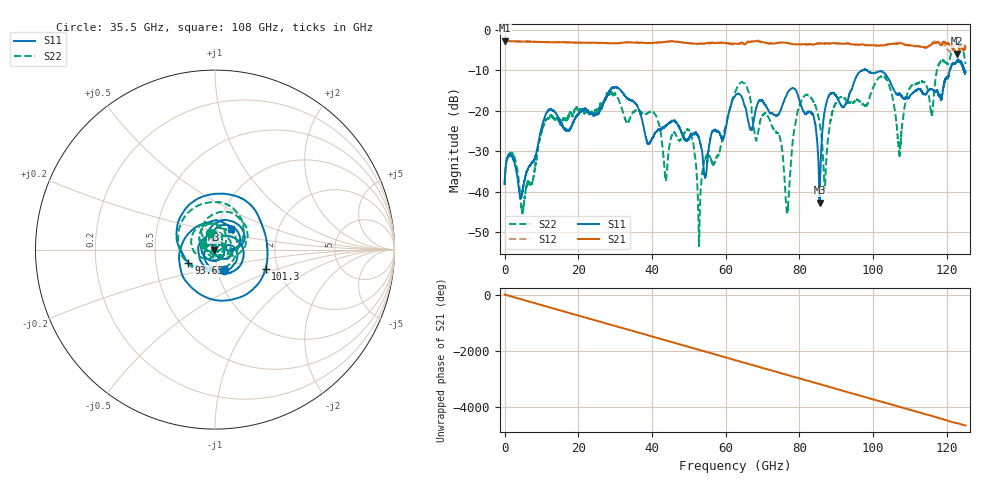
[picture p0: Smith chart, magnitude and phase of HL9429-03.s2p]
! 1/9/2024 4:34:33 PM
! H:\PROTOTYPE_DATA\110GHZ-ATTN\3DB\3089.S2P
! CHANNEL.1
! TR.MEASUREMENT
! CORRECTED.DATA
# GHZ S RI R 50.0
! FREQ.GHZ  S11RE  S11IM  S21RE  S21IM  S12RE  S12IM  S22RE  S22IM
!; PortSelection: Port_12
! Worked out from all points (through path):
!   5000 points, 25 MHz to 125 GHz, reference 50 ohm
!   highest |S21| = -2.70 dB at 25 MHz (marker M1); lowest = -5.9 dB at 122.8 GHz (marker M2)
!   group delay of S21, straight-line fit = 104 ps
!   lowest |S11| = -42.7 dB at 85.45 GHz (marker M3), VSWR 1.01, Z = 49.3 - j0.0201 ohm
!   |S11| at or under -10 dB: start of sweep to 97.18 GHz; 98.2 GHz to 120.8 GHz (22.57 GHz wide, 20.6 % of centre); 124.5879 GHz to end of sweep
!   |S22| runs from -53.5 to -2.9 dB; largest |S21 - S12| = 0.23
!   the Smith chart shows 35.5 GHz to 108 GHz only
!   S11 on the Smith chart (normalised r, x): 35.5 GHz: 1.08, -0.25; 93.65 GHz: 0.74, -0.11; 101.3 GHz: 1.72, -0.41; 108 GHz: 1.16, +0.27
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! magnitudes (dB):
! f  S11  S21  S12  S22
! 25 MHz  -38.2  -2.7  -2.7  -38.2
! 4.925 GHz  -39.8  -2.9  -2.9  -45.2
! 11.2 GHz  -20.9  -3.1  -3.1  -22.3
! 20.88 GHz  -20.3  -3.2  -3.2  -19.7
! 35.5 GHz  -18.2  -3.2  -3.2  -20.0
! 41.7 GHz  -24.7  -3.1  -3.2  -22.8
! 43.73 GHz  -23.9  -3.0  -3.0  -37.4
! 50.27 GHz  -26.3  -3.4  -3.2  -24.9
! 52.88 GHz  -27.2  -3.4  -3.5  -49.5
! 62.52 GHz  -16.3  -3.4  -3.5  -15.5
! 74.33 GHz  -20.9  -3.3  -3.2  -25.8
! 76.65 GHz  -15.8  -3.3  -3.4  -45.4
! 79.55 GHz  -16.2  -3.6  -3.6  -20.1
! 83.35 GHz  -20.7  -3.6  -3.6  -17.1
! 85.45 GHz  -42.7  -3.4  -3.4  -23.0
! 86.9 GHz  -19.7  -3.4  -3.3  -39.5
! 93.65 GHz  -15.6  -3.5  -3.6  -18.0
! 101.3 GHz  -10.4  -4.0  -3.9  -12.1
! 104.2 GHz  -12.2  -3.6  -3.6  -13.4
! 108 GHz  -16.8  -3.5  -3.5  -22.6
! 122.8 GHz  -7.8  -5.9  -3.4  -3.1
! 125 GHz  -10.4  -4.2  -4.1  -8.5
